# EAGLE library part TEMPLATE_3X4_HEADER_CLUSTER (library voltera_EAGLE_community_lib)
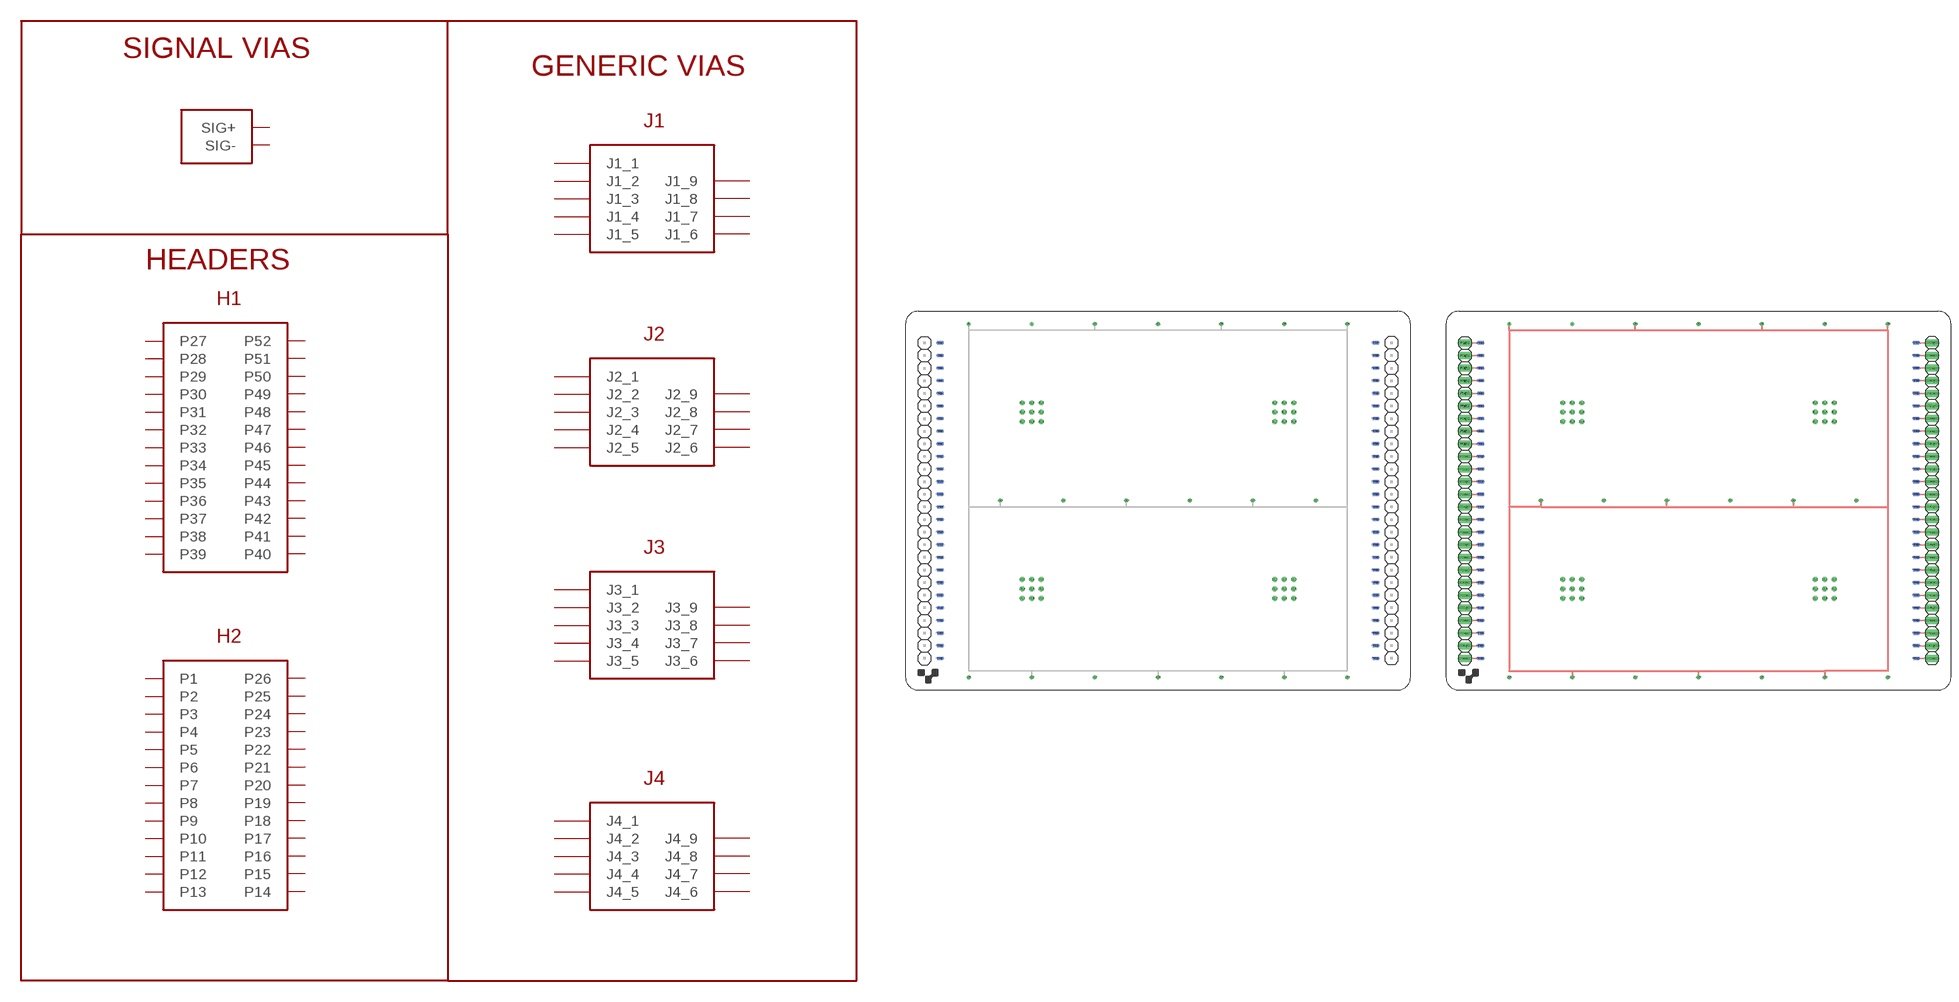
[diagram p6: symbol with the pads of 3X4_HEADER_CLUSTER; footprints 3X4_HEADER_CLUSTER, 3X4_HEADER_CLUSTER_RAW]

Designator prefix -

## TEMPLATE_3X4_HEADER_CLUSTER_TEMPLATE  [3X4_HEADER_CLUSTER]
+  SIG+
+@1  SIG+
+@2  SIG+
+@3  SIG+
+@4  SIG+
+@5  SIG+
+@6  SIG+
+@7  SIG+
+@8  SIG+
+@9  SIG+
-  SIG-
-@1  SIG-
-@2  SIG-
-@3  SIG-
-@4  SIG-
-@5  SIG-
-@6  SIG-
-@7  SIG-
-@8  SIG-
-@9  SIG-
J1_1  J1_1
J1_2  J1_2
J1_3  J1_3
J1_4  J1_4
J1_5  J1_5
J1_6  J1_6
J1_7  J1_7
J1_8  J1_8
J1_9  J1_9
J2_1  J2_1
J2_2  J2_2
J2_3  J2_3
J2_4  J2_4
J2_5  J2_5
J2_6  J2_6
J2_7  J2_7
J2_8  J2_8
J2_9  J2_9
J3_1  J3_1
J3_2  J3_2
J3_3  J3_3
J3_4  J3_4
J3_5  J3_5
J3_6  J3_6
J3_7  J3_7
J3_8  J3_8
J3_9  J3_9
J4_1  J4_1
J4_2  J4_2
J4_3  J4_3
J4_4  J4_4
J4_5  J4_5
J4_6  J4_6
J4_7  J4_7
J4_8  J4_8
J4_9  J4_9
P1  P1
P1@1  P1
P2  P2
P2@1  P2
P3  P3
P3@1  P3
P4  P4
P4@1  P4
P5  P5
P5@1  P5
P6  P6
P6@1  P6
P7  P7
P7@1  P7
P8  P8
P8@1  P8
P9  P9
P9@1  P9
P10  P10
P10@1  P10
P11  P11
P11@1  P11
P12  P12
P12@1  P12
P13  P13
P13@1  P13
P14  P14
P14@1  P14
P15  P15
P15@1  P15
P16  P16
P16@1  P16
P17  P17
P17@1  P17
P18  P18
P18@1  P18
P19  P19
P19@1  P19
P20  P20
P20@1  P20
P21  P21
P21@1  P21
P22  P22
P22@1  P22
P23  P23
P23@1  P23
P24  P24
P24@1  P24
P25  P25
P25@1  P25
P26  P26
P26@1  P26
P27  P27
P27@1  P27
P28  P28
P28@1  P28
P29  P29
P29@1  P29
P30  P30
P30@1  P30
P31  P31
P31@1  P31
P32  P32
P32@1  P32
P33  P33
P33@1  P33
P34  P34
P34@1  P34
P35  P35
P35@1  P35
P36  P36
P36@1  P36
P37  P37
P37@1  P37
P38  P38
P38@1  P38
P39  P39
P39@1  P39
P40  P40
P40@1  P40
P41  P41
P41@1  P41
P42  P42
P42@1  P42
P43  P43
P43@1  P43
P44  P44
P44@1  P44
P45  P45
P45@1  P45
P46  P46
P46@1  P46
P47  P47
P47@1  P47
P48  P48
P48@1  P48
P49  P49
P49@1  P49
P50  P50
P50@1  P50
P51  P51
P51@1  P51
P52  P52
P52@1  P52

## TEMPLATE_3X4_HEADER_CLUSTER_RAW  [3X4_HEADER_CLUSTER_RAW]
+  SIG+
+@1  SIG+
+@2  SIG+
+@3  SIG+
+@4  SIG+
+@5  SIG+
+@6  SIG+
+@7  SIG+
+@8  SIG+
+@9  SIG+
-  SIG-
-@1  SIG-
-@2  SIG-
-@3  SIG-
-@4  SIG-
-@5  SIG-
-@6  SIG-
-@7  SIG-
-@8  SIG-
-@9  SIG-
J1_1  J1_1
J1_2  J1_2
J1_3  J1_3
J1_4  J1_4
J1_5  J1_5
J1_6  J1_6
J1_7  J1_7
J1_8  J1_8
J1_9  J1_9
J2_1  J2_1
J2_2  J2_2
J2_3  J2_3
J2_4  J2_4
J2_5  J2_5
J2_6  J2_6
J2_7  J2_7
J2_8  J2_8
J2_9  J2_9
J3_1  J3_1
J3_2  J3_2
J3_3  J3_3
J3_4  J3_4
J3_5  J3_5
J3_6  J3_6
J3_7  J3_7
J3_8  J3_8
J3_9  J3_9
J4_1  J4_1
J4_2  J4_2
J4_3  J4_3
J4_4  J4_4
J4_5  J4_5
J4_6  J4_6
J4_7  J4_7
J4_8  J4_8
J4_9  J4_9
P1  P1
P1@1  P1
P1@2  P1
P2  P2
P2@1  P2
P2@2  P2
P3  P3
P3@1  P3
P3@2  P3
P4  P4
P4@1  P4
P4@2  P4
P5  P5
P5@1  P5
P5@2  P5
P6  P6
P6@1  P6
P6@2  P6
P7  P7
P7@1  P7
P7@2  P7
P8  P8
P8@1  P8
P8@2  P8
P9  P9
P9@1  P9
P9@2  P9
P10  P10
P10@1  P10
P10@2  P10
P11  P11
P11@1  P11
P11@2  P11
P12  P12
P12@1  P12
P12@2  P12
P13  P13
P13@1  P13
P13@2  P13
P14  P14
P14@1  P14
P14@2  P14
P15  P15
P15@1  P15
P15@2  P15
P16  P16
P16@1  P16
P16@2  P16
P17  P17
P17@1  P17
P17@2  P17
P18  P18
P18@1  P18
P18@2  P18
P19  P19
P19@1  P19
P19@2  P19
P20  P20
P20@1  P20
P20@2  P20
P21  P21
P21@1  P21
P21@2  P21
P22  P22
P22@1  P22
P22@2  P22
P23  P23
P23@1  P23
P23@2  P23
P24  P24
P24@1  P24
P24@2  P24
P25  P25
P25@1  P25
P25@2  P25
P26  P26
P26@1  P26
P26@2  P26
P27  P27
P27@1  P27
P27@2  P27
P28  P28
P28@1  P28
P28@2  P28
P29  P29
P29@1  P29
P29@2  P29
P30  P30
P30@1  P30
P30@2  P30
P31  P31
P31@1  P31
P31@2  P31
P32  P32
P32@1  P32
P32@2  P32
P33  P33
P33@1  P33
P33@2  P33
P34  P34
P34@1  P34
P34@2  P34
P35  P35
P35@1  P35
P35@2  P35
P36  P36
P36@1  P36
P36@2  P36
P37  P37
P37@1  P37
P37@2  P37
P38  P38
P38@1  P38
P38@2  P38
P39  P39
P39@1  P39
P39@2  P39
P40  P40
P40@1  P40
P40@2  P40
P41  P41
P41@1  P41
P41@2  P41
P42  P42
P42@1  P42
P42@2  P42
P43  P43
P43@1  P43
P43@2  P43
P44  P44
P44@1  P44
P44@2  P44
P45  P45
P45@1  P45
P45@2  P45
P46  P46
P46@1  P46
P46@2  P46
P47  P47
P47@1  P47
P47@2  P47
P48  P48
P48@1  P48
P48@2  P48
P49  P49
P49@1  P49
P49@2  P49
P50  P50
P50@1  P50
P50@2  P50
P51  P51
P51@1  P51
P51@2  P51
P52  P52
P52@1  P52
P52@2  P52

## Footprint 3X4_HEADER_CLUSTER (pad centres in mm)
drill 0.3 pad 0.8: + 12.7,73.66; +@1 38.1,73.66; +@2 63.5,73.66; +@3 19.05,38.1; +@4 44.45,38.1; +@5 69.85,38.1; +@6 88.9,73.66; +@7 25.4,2.54; +@8 50.8,2.54; +@9 76.2,2.54; - 25.4,73.66; -@1 50.8,73.66; -@2 76.2,73.66; -@3 82.55,38.1; -@4 57.15,38.1; -@5 31.75,38.1; -@6 12.7,2.54; -@7 38.1,2.54; -@8 63.5,2.54; -@9 88.9,2.54
drill 0.3 pad 1: J1_1 23.495,57.785; J1_2 25.4,57.785; J1_3 27.305,57.785; J1_4 23.495,55.88; J1_5 25.4,55.88; J1_6 27.305,55.88; J1_7 23.495,53.975; J1_8 25.4,53.975; J1_9 27.305,53.975; J2_1 76.2,57.785; J2_2 74.295,57.785; J2_3 78.105,57.785; J2_4 74.295,55.88; J2_5 76.2,55.88; J2_6 78.105,55.88; J2_7 74.295,53.975; J2_8 76.2,53.975; J2_9 78.105,53.975; J3_1 74.295,22.225; J3_2 76.2,22.225; J3_3 78.105,22.225; J3_4 74.295,20.32; J3_5 76.2,20.32; J3_6 78.105,20.32; J3_7 74.295,18.415; J3_8 76.2,18.415; J3_9 78.105,18.415; J4_1 23.495,22.225; J4_2 25.4,22.225; J4_3 27.305,22.225; J4_4 23.495,20.32; J4_5 25.4,20.32; J4_6 27.305,20.32; J4_7 23.495,18.415; J4_8 25.4,18.415; J4_9 27.305,18.415
smd 1.27 x 0.635: P1 6.985,69.85; P2 6.985,67.31; P3 6.985,64.77; P4 6.985,62.23; P5 6.985,59.69; P6 6.985,57.15; P7 6.985,54.61; P8 6.985,52.07; P9 6.985,49.53; P10 6.985,46.99; P11 6.985,44.45; P12 6.985,41.91; P13 6.985,39.37; P14 6.985,36.83; P15 6.985,34.29; P16 6.985,31.75; P17 6.985,29.21; P18 6.985,26.67; P19 6.985,24.13; P20 6.985,21.59; P21 6.985,19.05; P22 6.985,16.51; P23 6.985,13.97; P24 6.985,11.43; P25 6.985,8.89; P26 6.985,6.35; P27 94.615,69.85; P28 94.615,67.31; P29 94.615,64.77; P30 94.615,62.23; P31 94.615,59.69; P32 94.615,57.15; P33 94.615,54.61; P34 94.615,52.07; P35 94.615,49.53; P36 94.615,46.99; P37 94.615,44.45; P38 94.615,41.91; P39 94.615,39.37; P40 94.615,36.83; P41 94.615,34.29; P42 94.615,31.75; P43 94.615,29.21; P44 94.615,26.67; P45 94.615,24.13; P46 94.615,21.59; P47 94.615,19.05; P48 94.615,16.51; P49 94.615,13.97; P50 94.615,11.43; P51 94.615,8.89; P52 94.615,6.35
smd 1.27 x 0.635 bottom: P1@1 6.985,69.85; P2@1 6.985,67.31; P3@1 6.985,64.77; P4@1 6.985,62.23; P5@1 6.985,59.69; P6@1 6.985,57.15; P7@1 6.985,54.61; P8@1 6.985,52.07; P9@1 6.985,49.53; P10@1 6.985,46.99; P11@1 6.985,44.45; P12@1 6.985,41.91; P13@1 6.985,39.37; P14@1 6.985,36.83; P15@1 6.985,34.29; P16@1 6.985,31.75; P17@1 6.985,29.21; P18@1 6.985,26.67; P19@1 6.985,24.13; P20@1 6.985,21.59; P21@1 6.985,19.05; P22@1 6.985,16.51; P23@1 6.985,13.97; P24@1 6.985,11.43; P25@1 6.985,8.89; P26@1 6.985,6.35; P27@1 94.615,69.85; P28@1 94.615,67.31; P29@1 94.615,64.77; P30@1 94.615,62.23; P31@1 94.615,59.69; P32@1 94.615,57.15; P33@1 94.615,54.61; P34@1 94.615,52.07; P35@1 94.615,49.53; P36@1 94.615,46.99; P37@1 94.615,44.45; P38@1 94.615,41.91; P39@1 94.615,39.37; P40@1 94.615,36.83; P41@1 94.615,34.29; P42@1 94.615,31.75; P43@1 94.615,29.21; P44@1 94.615,26.67; P45@1 94.615,24.13; P46@1 94.615,21.59; P47@1 94.615,19.05; P48@1 94.615,16.51; P49@1 94.615,13.97; P50@1 94.615,11.43; P51@1 94.615,8.89; P52@1 94.615,6.35

## Footprint 3X4_HEADER_CLUSTER_RAW (pad centres in mm)
drill 0.3 pad 0.8: + 12.7,73.66; +@1 38.1,73.66; +@2 63.5,73.66; +@3 19.05,38.1; +@4 44.45,38.1; +@5 69.85,38.1; +@6 88.9,73.66; +@7 25.4,2.54; +@8 50.8,2.54; +@9 76.2,2.54; - 25.4,73.66; -@1 50.8,73.66; -@2 76.2,73.66; -@3 82.55,38.1; -@4 57.15,38.1; -@5 31.75,38.1; -@6 12.7,2.54; -@7 38.1,2.54; -@8 63.5,2.54; -@9 88.9,2.54
drill 0.3 pad 1: J1_1 23.495,57.785; J1_2 25.4,57.785; J1_3 27.305,57.785; J1_4 23.495,55.88; J1_5 25.4,55.88; J1_6 27.305,55.88; J1_7 23.495,53.975; J1_8 25.4,53.975; J1_9 27.305,53.975; J2_1 76.2,57.785; J2_2 74.295,57.785; J2_3 78.105,57.785; J2_4 74.295,55.88; J2_5 76.2,55.88; J2_6 78.105,55.88; J2_7 74.295,53.975; J2_8 76.2,53.975; J2_9 78.105,53.975; J3_1 74.295,22.225; J3_2 76.2,22.225; J3_3 78.105,22.225; J3_4 74.295,20.32; J3_5 76.2,20.32; J3_6 78.105,20.32; J3_7 74.295,18.415; J3_8 76.2,18.415; J3_9 78.105,18.415; J4_1 23.495,22.225; J4_2 25.4,22.225; J4_3 27.305,22.225; J4_4 23.495,20.32; J4_5 25.4,20.32; J4_6 27.305,20.32; J4_7 23.495,18.415; J4_8 25.4,18.415; J4_9 27.305,18.415
smd 1.27 x 0.635: P1 6.985,69.85; P2 6.985,67.31; P3 6.985,64.77; P4 6.985,62.23; P5 6.985,59.69; P6 6.985,57.15; P7 6.985,54.61; P8 6.985,52.07; P9 6.985,49.53; P10 6.985,46.99; P11 6.985,44.45; P12 6.985,41.91; P13 6.985,39.37; P14 6.985,36.83; P15 6.985,34.29; P16 6.985,31.75; P17 6.985,29.21; P18 6.985,26.67; P19 6.985,24.13; P20 6.985,21.59; P21 6.985,19.05; P22 6.985,16.51; P23 6.985,13.97; P24 6.985,11.43; P25 6.985,8.89; P26 6.985,6.35; P27 94.615,69.85; P28 94.615,67.31; P29 94.615,64.77; P30 94.615,62.23; P31 94.615,59.69; P32 94.615,57.15; P33 94.615,54.61; P34 94.615,52.07; P35 94.615,49.53; P36 94.615,46.99; P37 94.615,44.45; P38 94.615,41.91; P39 94.615,39.37; P40 94.615,36.83; P41 94.615,34.29; P42 94.615,31.75; P43 94.615,29.21; P44 94.615,26.67; P45 94.615,24.13; P46 94.615,21.59; P47 94.615,19.05; P48 94.615,16.51; P49 94.615,13.97; P50 94.615,11.43; P51 94.615,8.89; P52 94.615,6.35
smd 1.27 x 0.635 bottom: P1@1 6.985,69.85; P2@1 6.985,67.31; P3@1 6.985,64.77; P4@1 6.985,62.23; P5@1 6.985,59.69; P6@1 6.985,57.15; P7@1 6.985,54.61; P8@1 6.985,52.07; P9@1 6.985,49.53; P10@1 6.985,46.99; P11@1 6.985,44.45; P12@1 6.985,41.91; P13@1 6.985,39.37; P14@1 6.985,36.83; P15@1 6.985,34.29; P16@1 6.985,31.75; P17@1 6.985,29.21; P18@1 6.985,26.67; P19@1 6.985,24.13; P20@1 6.985,21.59; P21@1 6.985,19.05; P22@1 6.985,16.51; P23@1 6.985,13.97; P24@1 6.985,11.43; P25@1 6.985,8.89; P26@1 6.985,6.35; P27@1 94.615,69.85; P28@1 94.615,67.31; P29@1 94.615,64.77; P30@1 94.615,62.23; P31@1 94.615,59.69; P32@1 94.615,57.15; P33@1 94.615,54.61; P34@1 94.615,52.07; P35@1 94.615,49.53; P36@1 94.615,46.99; P37@1 94.615,44.45; P38@1 94.615,41.91; P39@1 94.615,39.37; P40@1 94.615,36.83; P41@1 94.615,34.29; P42@1 94.615,31.75; P43@1 94.615,29.21; P44@1 94.615,26.67; P45@1 94.615,24.13; P46@1 94.615,21.59; P47@1 94.615,19.05; P48@1 94.615,16.51; P49@1 94.615,13.97; P50@1 94.615,11.43; P51@1 94.615,8.89; P52@1 94.615,6.35
drill 1.016 long: P1@2 3.81,69.85; P2@2 3.81,67.31; P3@2 3.81,64.77; P4@2 3.81,62.23; P5@2 3.81,59.69; P6@2 3.81,57.15; P7@2 3.81,54.61; P8@2 3.81,52.07; P9@2 3.81,49.53; P10@2 3.81,46.99; P11@2 3.81,44.45; P12@2 3.81,41.91; P13@2 3.81,39.37; P14@2 3.81,36.83; P15@2 3.81,34.29; P16@2 3.81,31.75; P17@2 3.81,29.21; P18@2 3.81,26.67; P19@2 3.81,24.13; P20@2 3.81,21.59; P21@2 3.81,19.05; P22@2 3.81,16.51; P23@2 3.81,13.97; P24@2 3.81,11.43; P25@2 3.81,8.89; P26@2 3.81,6.35; P27@2 97.79,69.85; P28@2 97.79,67.31; P29@2 97.79,64.77; P30@2 97.79,62.23; P31@2 97.79,59.69; P32@2 97.79,57.15; P33@2 97.79,54.61; P34@2 97.79,52.07; P35@2 97.79,49.53; P36@2 97.79,46.99; P37@2 97.79,44.45; P38@2 97.79,41.91; P39@2 97.79,39.37; P40@2 97.79,36.83; P41@2 97.79,34.29; P42@2 97.79,31.75; P43@2 97.79,29.21; P44@2 97.79,26.67; P45@2 97.79,24.13; P46@2 97.79,21.59; P47@2 97.79,19.05; P48@2 97.79,16.51; P49@2 97.79,13.97; P50@2 97.79,11.43; P51@2 97.79,8.89; P52@2 97.79,6.35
